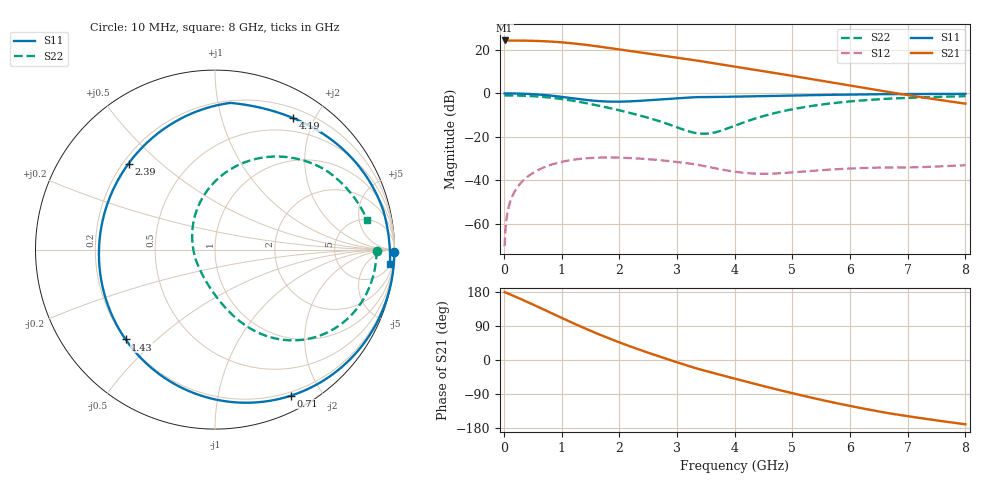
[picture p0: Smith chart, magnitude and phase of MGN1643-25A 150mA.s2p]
! Port[1] = GATE
! Port[2] = DRAIN
! [Type]  S-parameter s2p file touchstone ver. 1.0
! [Object]  MGN1643-25A
! [Bias]  150 mA
! [Version]  1.0
! [Date]  Tue May 19 13:03:48 2026
! [Source]  This file was created in JSC "ICC Milandr".
! [Disclaimer] Property of JSC "ICC Milandr". Unauthorized reproduction and/or distribution is strictly prohibited.
!  The file and the data are provided "AS IS" and with all faults and disclaim all warranties, express and implied, including
!  without limitation any implied warranties of merchantability, fitness for a particular purpose.
!  JSC "ICC Milandr" assumes no liability for:
!  1) the accuracy of the data provided;
!  2) the proper functioning of this data;
!  3) infringement of patents, copyrights or intellectual property rights resulting from the use of this data.
!  JSC "ICC Milandr" reserves the right to make changes to the products and the data without prior notice.
!  Please, be aware that your receipt and use of the file provided shall serve as acceptance of these terms and conditions.
!  If you do not accept these terms, you should return or destroy this file and any other accompanying information immediately.
# Hz S MA R 12.5
! freq  S11mag  S11ang  S21mag  S21ang  S12mag  S12ang  S22mag  S22ang
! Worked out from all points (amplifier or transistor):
!   800 points, 10 MHz to 8 GHz, reference 12.5 ohm
!   highest |S21| = 24.4 dB at 10 MHz (marker M1)
!   |S21| within 3 dB of that: start of sweep to 1.699 GHz
!   unconditionally stable (mu >= 1): 2.474 GHz to 6.581 GHz
!   at 1.34 GHz: K = 0.51, MSG = 26.3 dB, |S12| = -30.0 dB
!   at 4.01 GHz: K = 2.07, MAG = 18.3 dB, |S12| = -36.1 dB
!   at 8 GHz: K = 0.57, MSG = 14.2 dB, |S12| = -33.0 dB
!   S11 on the Smith chart (normalised r, x): 10 MHz: open; 710 MHz: 0.16, -1.64; 1.43 GHz: 0.20, -0.40; 2.39 GHz: 0.22, +0.39; 4.19 GHz: 0.32, +1.71; 8 GHz: 6, -23
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1e7  0.9998 -0.8  16.55 179.2  0.0003057 82.3  0.9 -0.4
1.2e8  0.9985 -10.2  16.49 172.2  0.003619 82.5  0.8987 -4.9
3.6e8  0.9821 -30.8  16.38 156.1  0.01076 68.8  0.8826 -14.8
5.3e8  0.9568 -45.9  16.19 144.4  0.0156 58.5  0.8593 -21.9
7.1e8  0.9174 -62.5  15.86 131.7  0.02034 47.4  0.8232 -29.4
8.7e8  0.873 -77.7  15.42 120.3  0.02407 37.4  0.7819 -35.8
1.02e9  0.8265 -92.5  14.9 109.7  0.02704 28.1  0.7366 -41.7
1.18e9  0.7759 -108.8  14.24 98.5  0.02958 18.3  0.6834 -47.6
1.35e9  0.7264 -126.5  13.45 87.0  0.03155 8.3  0.6239 -53.5
1.43e9  0.7061 -134.9  13.06 81.7  0.03222 3.7  0.5957 -56.1
1.65e9  0.6644 -158.0  11.96 67.5  0.03334 -8.4  0.5195 -62.7
1.88e9  0.646 178.8  10.84 53.5  0.03351 -20.2  0.4447 -69.0
2.12e9  0.6517 156.6  9.743 39.7  0.03287 -31.7  0.3737 -75.3
2.39e9  0.6795 135.2  8.635 25.0  0.03144 -43.7  0.3019 -83.0
2.68e9  0.7219 116.1  7.596 9.9  0.02931 -55.8  0.2327 -93.5
3.32e9  0.8192 84.8  5.777 -21.5  0.02327 -79.9  0.1228 -147.3
4.01e9  0.8429 64.0  4.123 -49.6  0.01575 -75.9  0.1827 132.3
4.19e9  0.852 59.4  3.779 -56.7  0.01477 -71.9  0.2234 119.5
4.76e9  0.8837 46.5  2.858 -78.7  0.01452 -58.6  0.3705 91.3
5.34e9  0.914 35.0  2.131 -99.7  0.01656 -54.0  0.5165 70.8
6.67e9  0.9628 13.0  1.078 -140.5  0.01982 -63.0  0.7577 36.0
8e9  0.9781 -4.6  0.5816 -169.7  0.02226 -84.6  0.8634 11.2
